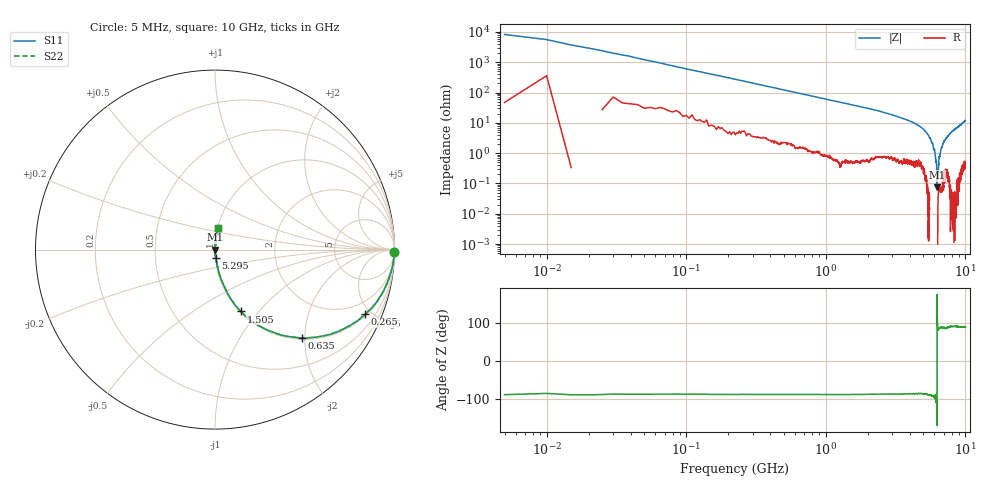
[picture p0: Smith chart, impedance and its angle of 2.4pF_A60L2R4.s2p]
! Amotech Co.,Ltd.
! http://www.amotech.co.kr/
! Part Number: A60L2R4
! These Parameters are Measured in Series Mode Connection
! Operation Temp=25[degC], DC Bias Voltage=0[V]
! Freq. Start=5[MHz] Stop=10[GHz], 2000[Steps]
! Date: Monday, July 14, 2020, 09:29:32
# GHZ S RI R 50.000000
!Freq.(Hz) S11(Real) S11(Imag) S21(Real) S21(Imag) S12(Real) S12(Imag) S22(Real) S22(Imag)
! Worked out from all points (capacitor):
!   2000 points, 5 MHz to 10 GHz, reference 50 ohm
!   read as one part in series: C = 2.63 pF near 55 MHz
!   lowest |Z| = 75.8 mohm at 6.265 GHz (marker M1)
!   series resonance near 6.263 GHz, so ESL is about 250 pH
!   S11 on the Smith chart (normalised r, x): 5 MHz: open; 265 MHz: 1.10, -4.62; 635 MHz: 1.03, -1.93; 1.505 GHz: 1.01, -0.81; 5.295 GHz: 1.00, -0.09; 10 GHz: 1.01, +0.24
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0.005  0.9998 -0.0122  0.000219 0.0122  0.000219 0.0122  0.9998 -0.0122
0.065  0.9854 -0.104  0.0146 0.104  0.0146 0.104  0.9854 -0.104
0.1  0.9688 -0.1601  0.0312 0.1601  0.0312 0.1601  0.9688 -0.1601
0.265  0.837 -0.3592  0.163 0.3592  0.163 0.3592  0.837 -0.3592
0.635  0.4832 -0.492  0.5168 0.492  0.5168 0.492  0.4832 -0.492
1.005  0.2718 -0.4379  0.7282 0.4379  0.7282 0.4379  0.2718 -0.4379
1.505  0.1442 -0.3445  0.8558 0.3445  0.8558 0.3445  0.1442 -0.3445
1.675  0.1201 -0.3177  0.8799 0.3177  0.8799 0.3177  0.1201 -0.3177
3.34  0.0276 -0.1487  0.9724 0.1487  0.9724 0.1487  0.0276 -0.1487
5.005  0.00593 -0.0604  0.9941 0.0604  0.9941 0.0604  0.00593 -0.0604
5.295  0.00284 -0.0457  0.9972 0.0457  0.9972 0.0457  0.00284 -0.0457
5.82  -0.000786 -0.021  1.001 0.021  1.001 0.021  -0.000786 -0.021
6.015  -0.00162 -0.0125  1.002 0.0125  1.002 0.0125  -0.00162 -0.0125
6.18  -0.00166 -0.00521  1.002 0.00521  1.002 0.00521  -0.00166 -0.00521
6.265  -0.000754 8.29e-05  1.001 -8.29e-05  1.001 -8.29e-05  -0.000754 8.29e-05
6.305  -0.000281 0.00195  1 -0.00195  1 -0.00195  -0.000281 0.00195
6.48  0.000681 0.00688  0.9993 -0.00688  0.9993 -0.00688  0.000681 0.00688
6.67  0.000796 0.0121  0.9992 -0.0121  0.9992 -0.0121  0.000796 0.0121
6.9  0.00214 0.0201  0.9979 -0.0201  0.9979 -0.0201  0.00214 0.0201
7.275  0.00313 0.0309  0.9969 -0.0309  0.9969 -0.0309  0.00313 0.0309
8.335  0.00367 0.0595  0.9963 -0.0595  0.9963 -0.0595  0.00367 0.0595
10  0.0173 0.1177  0.9827 -0.1177  0.9827 -0.1177  0.0173 0.1177
